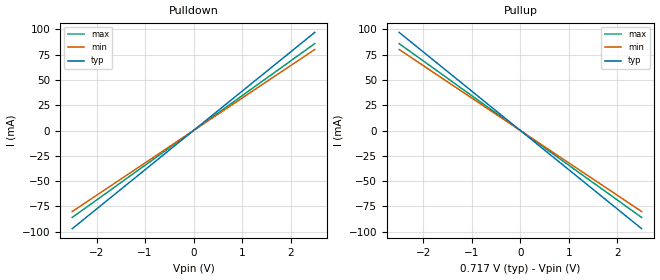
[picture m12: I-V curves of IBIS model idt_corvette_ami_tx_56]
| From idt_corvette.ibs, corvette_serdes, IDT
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|   model   idt_corvette_ami_tx_56
[Model] idt_corvette_ami_tx_56
Model_type Output
C_comp 400f 400f 400f
Cref = 0
[Model Spec]
Vmeas 0. 0. 0.
Vref 0. 0. 0.
[Temperature Range]  25 100 0
[Voltage Range] .717 .697 .733
[Algorithmic Model]
Executable Windows_VisualStudio5_32 idt_corvette_tx.dll   idt_corvette_tx.ami
Executable Windows_ver_64   idt_corvette_tx_64.dll   idt_corvette_tx.ami
Executable Linux_gcc4.1.2_32   idt_corvette_tx.linux.so   idt_corvette_tx.ami
Executable Linux_gcc3.2.3_64   idt_corvette_tx_64.linux.so idt_corvette_tx.ami
[End Algorithmic Model]
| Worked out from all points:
|   slope of the pulldown table from 0 to 0.108 V, typ, clamps not added: 25.8 ohm
|   slope of the pullup table from 0 to 0.108 V, typ, clamps not added: 25.8 ohm
[Pulldown]
-2.5V     -96.98mA   -80.07mA   -85.88mA
0V        0A         0A         0A
2.5V      96.98mA    80.07mA    85.88mA
[Pullup]
-2.5V     96.98mA    80.07mA    85.88mA
0V        0A         0A         0A
2.5V      -96.98mA   -80.07mA   -85.88mA
[Ramp]
dV/dt_r .284/14.436p .257/17.484p .278/16.302p
dV/dt_f .284/14.436p .257/17.484p .278/16.302p
